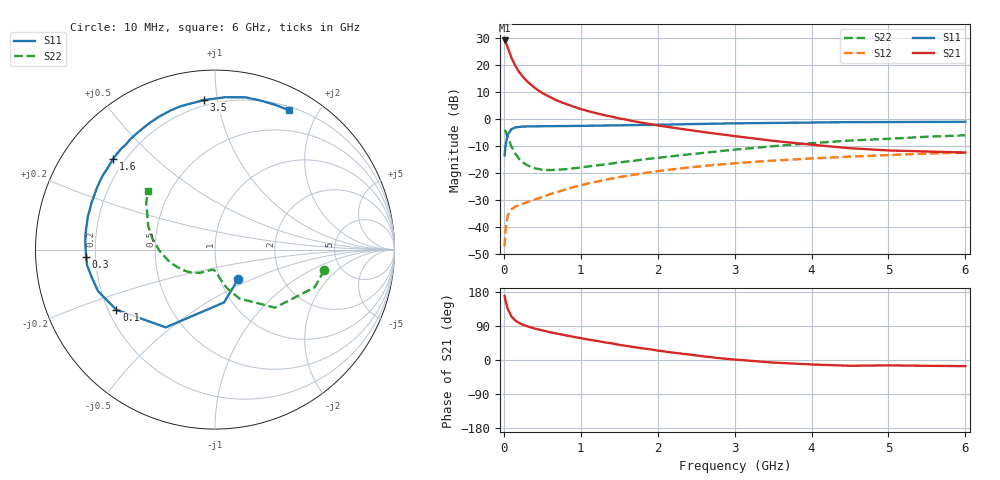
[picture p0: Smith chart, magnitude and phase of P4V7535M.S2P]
! SIEMENS Small Signal Semiconductors
! BFP182
! Si NPN RF Bipolar Junction Transistor in SOT143
! VCE = 0.75 V  IC = 35 mA
! Common Emitter S-Parameters:  March  1996
# GHz  S  MA  R  50
!  f  S11  S21  S12  S22
! GHz  MAG  ANG  MAG  ANG  MAG  ANG  MAG  ANG
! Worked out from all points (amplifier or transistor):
!   36 points, 10 MHz to 6 GHz, reference 50 ohm
!   highest |S21| = 28.9 dB at 10 MHz (marker M1)
!   |S21| within 3 dB of that: start of sweep to 55.79 MHz
!   unconditionally stable (mu >= 1): start of sweep to 32.58 MHz; 133 MHz to end of sweep
!   at 250 MHz: K = 1.48, MAG = 19.3 dB, |S12| = -31.4 dB
!   at 1.4 GHz: K = 2.51, MAG = 4.6 dB, |S12| = -22.1 dB
!   at 6 GHz: K = 1.92, MAG = -5.5 dB, |S12| = -12.5 dB
!   S11 on the Smith chart (normalised r, x): 10 MHz: 1.22, -0.42; 100 MHz: 0.23, -0.27; 300 MHz: 0.16, -0.03; 1.6 GHz: 0.16, +0.37; 3.5 GHz: 0.17, +0.92; 6 GHz: 0.24, +1.64
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0.01  0.2096 -52.0  28.02 169.2  0.0044 66.6  0.62 -10.5
0.02  0.2985 -80.3  26.88 159.0  0.0085 64.3  0.5933 -20.8
0.05  0.5126 -122.3  20.9 134.9  0.0164 50.8  0.4648 -44.1
0.1  0.6439 -148.6  13.29 114.4  0.0212 37.6  0.3039 -63.6
0.15  0.6915 -160.4  9.491 104.1  0.0239 35.5  0.2251 -72.6
0.2  0.705 -167.8  7.28 97.6  0.0251 36.7  0.1808 -77.9
0.25  0.718 -173.0  5.894 92.8  0.0268 38.0  0.1547 -81.7
0.3  0.7191 -176.6  4.947 89.3  0.0285 39.9  0.1388 -84.2
0.4  0.7227 177.8  3.732 83.0  0.032 44.8  0.1213 -88.6
0.5  0.7269 173.0  2.982 78.1  0.0358 47.3  0.1141 -92.6
0.6  0.7278 169.1  2.516 73.4  0.0402 49.7  0.1123 -96.0
0.7  0.7321 165.3  2.147 69.3  0.0444 51.6  0.1137 -98.9
0.8  0.7324 162.2  1.894 65.2  0.049 53.1  0.1167 -102.1
1.1  0.742 152.6  1.378 53.8  0.0641 54.5  0.1314 -111.9
1.3  0.7496 146.7  1.17 47.0  0.0731 54.0  0.1425 -118.2
1.6  0.7601 138.5  0.957 37.0  0.0879 52.5  0.1619 -126.6
2.2  0.7828 122.6  0.682 19.4  0.1163 47.1  0.2036 -144.1
2.8  0.8131 108.0  0.52 4.9  0.1422 40.1  0.2514 -161.8
3.5  0.8359 94.1  0.39 -6.8  0.168 31.7  0.3111 -179.2
4.5  0.8654 78.6  0.285 -15.2  0.1987 20.4  0.3951 160.5
5.5  0.8734 67.5  0.248 -15.3  0.2274 9.9  0.4645 145.7
6  0.8794 62.1  0.237 -16.2  0.2365 4.2  0.4938 138.8
